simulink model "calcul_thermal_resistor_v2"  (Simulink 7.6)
settings: Solver=ode15s  StartTime=0.0  StopTime=122  RelTol=1e-3
InitFcn:
  | clc
  | clear all
  | close all
  | Vcc=12;
  | R=1e3;
StopFcn:
  | close all
  | load Temp_Rth.mat
  | plotyy(x(1,:),x(2,:),x(1,:),x(3,:))
  | axis([0 140 25 55])
  | title('Température mesurée et résistance Rth')
  | xlabel('temps')
  | grid
libraries: fl_lib x19, nesl_utility x5, elec_lib x2

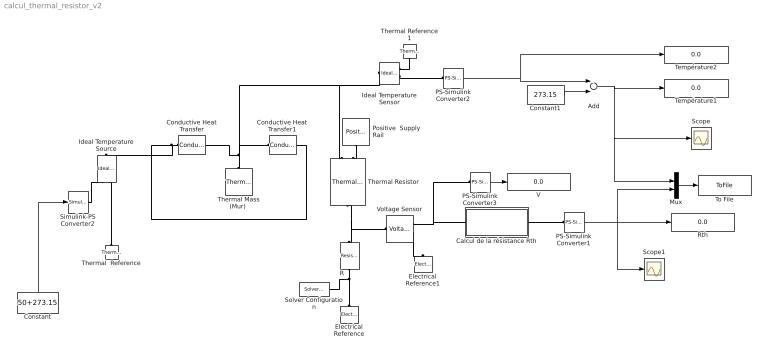
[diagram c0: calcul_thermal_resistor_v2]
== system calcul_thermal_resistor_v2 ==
  Add : Sum  Inputs=+-
  Calcul de la résistance Rth : Subsystem
  Conductive Heat Transfer : fl_lib/Thermal/Thermal Elements/Conductive Heat Transfer  DialogController=NetworkEngine.DynNeDlgSource  SystemSampleTime=-1  area=0.04 m^2  thickness=0.1 m  th_cond=46 W/(m*K)  Q_Log=off  T_Log=off  LocalVarNames=|Q|T  LocalVarDescs=|Q|T  LocalVarLogging=[0 0]
  Conductive Heat Transfer1 : fl_lib/Thermal/Thermal Elements/Conductive Heat Transfer  DialogController=NetworkEngine.DynNeDlgSource  SystemSampleTime=-1  area=0.04 m^2  thickness=0.1 m  th_cond=46 W/(m*K)  Q_Log=off  T_Log=off  LocalVarNames=|Q|T  LocalVarDescs=|Q|T  LocalVarLogging=[0 0]
  Constant : Constant  Value=50+273.15
  Constant1 : Constant  Value=273.15
  Electrical Reference : fl_lib/Electrical/Electrical Elements/Electrical Reference  DialogController=NetworkEngine.DynNeDlgSource  SystemSampleTime=-1  i_Log=off  LocalVarNames=|i  LocalVarDescs=|i  LocalVarLogging=[]
  Electrical Reference1 : fl_lib/Electrical/Electrical Elements/Electrical Reference  DialogController=NetworkEngine.DynNeDlgSource  SystemSampleTime=-1  i_Log=off  LocalVarNames=|i  LocalVarDescs=|i  LocalVarLogging=[]
  Ideal Temperature Sensor : fl_lib/Thermal/Thermal Sensors/Ideal Temperature Sensor  DialogController=NetworkEngine.DynNeDlgSource  SystemSampleTime=-1  Qs_Log=off  Ts_Log=off  LocalVarNames=|Qs|Ts  LocalVarDescs=|Qs|Ts  LocalVarLogging=[0 0]
  Ideal Temperature Source : fl_lib/Thermal/Thermal Sources/Ideal Temperature Source  DialogController=NetworkEngine.DynNeDlgSource  SystemSampleTime=-1  Q_Log=off  T_Log=off  LocalVarNames=|Q|T  LocalVarDescs=|Q|T  LocalVarLogging=[0 0]
  Mux : Mux  Inputs=2
  PS-Simulink Converter1 : nesl_utility/PS-Simulink Converter  DialogController=NetworkEngine.DynNeUtilDlgSource  SystemSampleTime=-1  PhysicalDomain=network_engine_domain  LeftPortType=input  RightPortType=output  SubClassName=ps_output  Unit=V  AffineConversion=off
  PS-Simulink Converter2 : nesl_utility/PS-Simulink Converter  DialogController=NetworkEngine.DynNeUtilDlgSource  SystemSampleTime=-1  PhysicalDomain=network_engine_domain  LeftPortType=input  RightPortType=output  SubClassName=ps_output  Unit=1  AffineConversion=off
  PS-Simulink Converter3 : nesl_utility/PS-Simulink Converter  DialogController=NetworkEngine.DynNeUtilDlgSource  SystemSampleTime=-1  PhysicalDomain=network_engine_domain  LeftPortType=input  RightPortType=output  SubClassName=ps_output  Unit=V  AffineConversion=off
  Positive  Supply Rail : elec_lib/Sources/Positive Supply Rail  DialogController=NetworkEngine.DynNeDlgSource  SystemSampleTime=-1  v0=Vcc V  current_Log=off  voltage_Log=off  power_Log=off  LocalVarNames=|current|voltage|power  LocalVarDescs=|Current (A)|Voltage (V)|Power (W)  LocalVarLogging=[0 0 0]
  R : fl_lib/Electrical/Electrical Elements/Resistor  DialogController=NetworkEngine.DynNeDlgSource  SystemSampleTime=-1  R=R Ohm  i_Log=off  v_Log=off  LocalVarNames=|current|voltage|power  LocalVarDescs=|Resistor current (A)|Voltage across resistor (V)|Power (W)  LocalVarLogging=[0 0 0]
  Rth : Display
  Scope : Scope
  Scope1 : Scope
  Simulink-PS Converter2 : nesl_utility/Simulink-PS Converter  DialogController=NetworkEngine.DynNeUtilDlgSource  SystemSampleTime=-1  PhysicalDomain=network_engine_domain  LeftPortType=input  RightPortType=output  SubClassName=ps_input  Unit=1  AffineConversion=off  InputFilterTimeConstant=.001  UdotUserProvided=0
  Solver Configuration : nesl_utility/Solver Configuration  DialogController=NetworkEngine.DynNeUtilDlgSource  SystemSampleTime=-1  PhysicalDomain=network_engine_domain  LeftPortType=input  RightPortType=generic  SubClassName=solver  Accelerate=off  Profile=off  ResidualTolerance=1e-9  MaxNonlinIter=12  MaxModeIter=2  DoFixedCost=off  UseLocalSampling=off  DoDC=off  LinearAlgebra=Sparse  LocalSolverSampleTime=.001  LocalSolverChoice=NE_BACKWARD_EULER_ADVANCER  UseLocalSolver=off
  Température1 : Display
  Température2 : Display
  Thermal  Reference : fl_lib/Thermal/Thermal Elements/Thermal Reference  DialogController=NetworkEngine.DynNeDlgSource  SystemSampleTime=-1  Q_Log=off  LocalVarNames=|Q  LocalVarDescs=|Q  LocalVarLogging=0
  "Thermal Mass (Mur) " : fl_lib/Thermal/Thermal Elements/Thermal Mass  DialogController=NetworkEngine.DynNeDlgSource  SystemSampleTime=-1  mass=1 kg  sp_heat=444 J/kg/K  init_temp=25 C  Q_Log=off  LocalVarNames=|heat_flow|temperature  LocalVarDescs=|Heat flow (J/s)|Mass temperature (K)  LocalVarLogging=[0 0]
  Thermal Reference1 : fl_lib/Thermal/Thermal Elements/Thermal Reference  DialogController=NetworkEngine.DynNeDlgSource  SystemSampleTime=-1  Q_Log=off  LocalVarNames=|Q  LocalVarDescs=|Q  LocalVarLogging=0
  Thermal Resistor : elec_lib/Passive Devices/Thermal Resistor  DialogController=NetworkEngine.DynNeDlgSource  SystemSampleTime=-1  R0=1 Ohm  T0=25 C  alpha=5e-05 1/K  tc=10 s  K_d=0.001 W/K  init_temp=25 C  current_Log=off  voltage_Log=off  power_Log=off  temperature_Log=off  heat_flow_Log=off  LocalVarNames=|current|voltage|power|temperature|heat_flow  LocalVarDescs=|Resistor current (A)|Voltage across resistor (V)|Power (W)|Themistor temperature (K)|Heat flow (J/s)  LocalVarLogging=[0 0 0 0 0]
  To File : ToFile  Filename=Temp_Rth  MatrixName=x
  V : Display
  Voltage Sensor : fl_lib/Electrical/Electrical Sensors/Voltage Sensor  DialogController=NetworkEngine.DynNeDlgSource  SystemSampleTime=-1  i1_Log=off  v1_Log=off  LocalVarNames=|i1|v1  LocalVarDescs=|i1|v1  LocalVarLogging=[]
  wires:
  Constant/1 -> Simulink-PS Converter2/1
  PS-Simulink Converter1/1 -> Scope1/1, Rth/1, Mux/2
  PS-Simulink Converter2/1 -> Add/1, Température2/1
  PS-Simulink Converter3/1 -> V/1
  Constant1/1 -> Add/2
  Add/1 -> Température1/1, Scope/1, Mux/1
  Mux/1 -> To File/1
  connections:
  Positive  Supply Rail/RConn1 -- Thermal Resistor/LConn2
  Thermal Resistor/RConn1 -- R/RConn1 -- Voltage Sensor/LConn1
  R/LConn1 -- Electrical Reference/LConn1 -- Solver Configuration/RConn1
  Voltage Sensor/RConn2 -- Electrical Reference1/LConn1
  Thermal  Reference/LConn1 -- Ideal Temperature Source/RConn2
  Simulink-PS Converter2/RConn1 -- Ideal Temperature Source/RConn1
  Conductive Heat Transfer/LConn1 -- Ideal Temperature Source/LConn1 -- Conductive Heat Transfer1/RConn1
  Thermal Reference1/LConn1 -- Ideal Temperature Sensor/RConn1
  Ideal Temperature Sensor/RConn2 -- PS-Simulink Converter2/LConn1
  Calcul de la résistance Rth/RConn1 -- PS-Simulink Converter1/LConn1
  Voltage Sensor/RConn1 -- Calcul de la résistance Rth/LConn1 -- PS-Simulink Converter3/LConn1
  "Thermal Mass (Mur) "/LConn1 -- Ideal Temperature Sensor/LConn1 -- Thermal Resistor/LConn1 -- Conductive Heat Transfer/RConn1 -- Conductive Heat Transfer1/LConn1

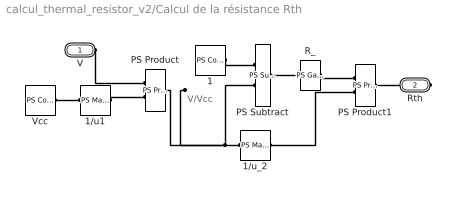
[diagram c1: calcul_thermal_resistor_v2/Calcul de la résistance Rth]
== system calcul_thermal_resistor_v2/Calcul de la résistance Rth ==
  note: V/Vcc
  1 : fl_lib/Physical Signals/Sources/PS Constant  DialogController=NetworkEngine.DynNeDlgSource  SystemSampleTime=-1  constant=1  LocalVarLogging=[]
  1/u1 : fl_lib/Physical Signals/Functions/PS Math Function  DialogController=NetworkEngine.DynNeDlgSource  SystemSampleTime=-1  fcn_choice=9  LocalVarLogging=[]
  1/u_2 : fl_lib/Physical Signals/Functions/PS Math Function  DialogController=NetworkEngine.DynNeDlgSource  SystemSampleTime=-1  fcn_choice=9  LocalVarLogging=[]
  PS Product : fl_lib/Physical Signals/Functions/PS Product  DialogController=NetworkEngine.DynNeDlgSource  SystemSampleTime=-1  LocalVarLogging=[]
  PS Product1 : fl_lib/Physical Signals/Functions/PS Product  DialogController=NetworkEngine.DynNeDlgSource  SystemSampleTime=-1  LocalVarLogging=[]
  PS Subtract : fl_lib/Physical Signals/Functions/PS Subtract  DialogController=NetworkEngine.DynNeDlgSource  SystemSampleTime=-1  LocalVarLogging=[]
  R_ : fl_lib/Physical Signals/Functions/PS Gain  DialogController=NetworkEngine.DynNeDlgSource  SystemSampleTime=-1  gain=R  LocalVarLogging=[]
  Vcc : fl_lib/Physical Signals/Sources/PS Constant  DialogController=NetworkEngine.DynNeDlgSource  SystemSampleTime=-1  constant=Vcc  LocalVarLogging=[]
  V : PMIOPort  Port=1  Side=Left
  Rth : PMIOPort  Port=2  Side=Right
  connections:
  1/RConn1 -- PS Subtract/LConn1
  Vcc/RConn1 -- 1/u1/LConn1
  1/u1/RConn1 -- PS Product/LConn2
  1/u_2/LConn1 -- PS Subtract/LConn2 -- PS Product/RConn1
  1/u_2/RConn1 -- PS Product1/LConn2
  R_/RConn1 -- PS Product1/LConn1
  PS Subtract/RConn1 -- R_/LConn1
  V/RConn1 -- PS Product/LConn1
  Rth/RConn1 -- PS Product1/RConn1
